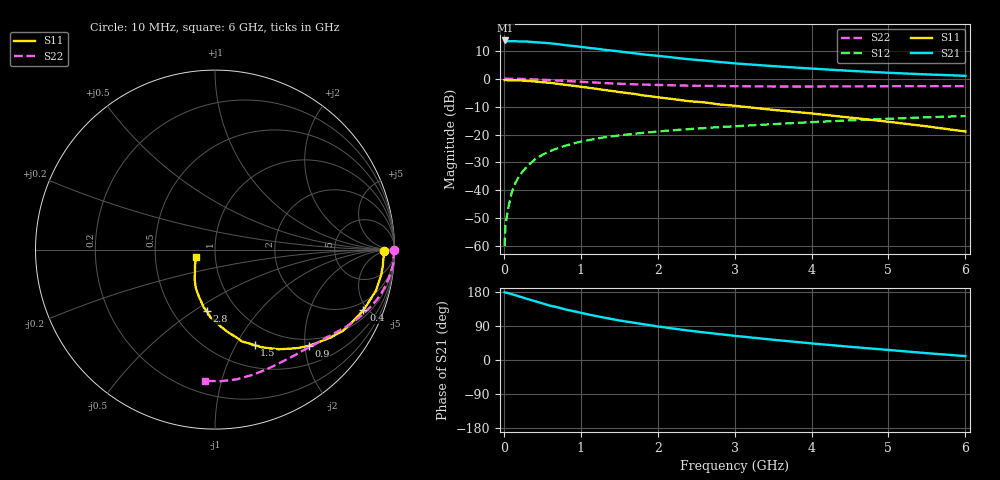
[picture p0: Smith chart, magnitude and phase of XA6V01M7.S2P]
! SIEMENS Discrete & RF Semiconductors
! BFY180
! Si NPN RF Bipolar Junction Transistor in MICRO-X
! VCE = 6 V  IC = 1.7 mA
! Common Emitter S-Parameters:  May  1997
# GHz  S  MA  R  50
!  f  S11  S21  S12  S22
! GHz  MAG  ANG  MAG  ANG  MAG  ANG  MAG  ANG
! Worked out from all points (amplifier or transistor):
!   36 points, 10 MHz to 6 GHz, reference 50 ohm
!   highest |S21| = 13.7 dB at 20 MHz (marker M1)
!   |S21| within 3 dB of that: start of sweep to 1.214 GHz
!   unconditionally stable (mu >= 1): 3.275 GHz to end of sweep
!   at 250 MHz: K = 0.09, MSG = 23.2 dB, |S12| = -33.1 dB
!   at 1.4 GHz: K = 0.60, MSG = 15.4 dB, |S12| = -20.7 dB
!   at 6 GHz: K = 1.06, MAG = 5.7 dB, |S12| = -13.4 dB
!   S11 on the Smith chart (normalised r, x): 10 MHz: 32, -5; 400 MHz: 1.41, -4.69; 900 MHz: 0.85, -2.08; 1.5 GHz: 0.75, -1.20; 2.8 GHz: 0.73, -0.57; 6 GHz: 0.81, -0.07
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0.01  0.9406 -0.5  4.725 178.7  0.001 72.7  0.9955 -0.2
0.02  0.9458 -1.1  4.839 178.0  0.0023 81.0  0.9999 -0.6
0.05  0.9394 -2.9  4.685 176.8  0.0043 88.2  0.9959 -1.5
0.1  0.9395 -5.5  4.703 173.9  0.0089 87.4  0.9961 -3.1
0.15  0.9367 -8.7  4.691 170.8  0.0136 84.6  0.9951 -4.7
0.3  0.9136 -16.8  4.628 161.4  0.0267 79.2  0.9813 -9.2
0.4  0.893 -22.2  4.501 155.5  0.0355 75.8  0.9717 -12.0
0.6  0.8441 -32.4  4.311 143.5  0.0503 69.3  0.9424 -17.4
0.7  0.8096 -37.2  4.159 139.0  0.057 66.0  0.927 -19.8
0.8  0.7755 -41.6  3.986 133.4  0.063 63.4  0.9094 -22.1
0.9  0.7485 -45.7  3.856 129.1  0.069 60.8  0.8948 -24.3
1.1  0.6888 -53.3  3.568 120.2  0.0791 56.7  0.8642 -28.2
1.2  0.6596 -57.3  3.446 115.9  0.0842 54.7  0.8508 -30.1
1.5  0.5768 -67.5  3.075 104.4  0.0965 49.8  0.8126 -35.0
1.9  0.4861 -78.4  2.644 91.8  0.1093 44.9  0.7779 -40.8
2.2  0.4309 -85.6  2.397 83.1  0.1192 42.1  0.761 -44.9
2.4  0.3961 -90.3  2.235 77.7  0.1247 40.3  0.7507 -47.5
2.8  0.3459 -97.5  1.993 68.3  0.1358 37.3  0.7385 -52.4
3.5  0.2762 -109.0  1.678 53.5  0.1534 32.3  0.727 -60.9
4.5  0.2012 -124.2  1.381 34.9  0.179 25.1  0.7286 -73.7
5.5  0.14 -142.7  1.192 18.0  0.2033 17.6  0.7339 -87.4
6  0.1132 -158.0  1.125 10.3  0.2144 13.4  0.7335 -94.3
